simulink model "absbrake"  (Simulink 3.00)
settings: Solver=ode45  SolverMode=SingleTasking  StartTime=0.0  StopTime=25  MaxStep=.01  RelTol=1e-3  AbsTol=1e-6
PreLoadFcn:
  | absdata
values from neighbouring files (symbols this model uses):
  ctrl = 1    [absdata.m]
  g = 32.18    [absdata.m]    (also in f14dat.m = 32.2; watergui.m = locdrawwater(hilim, lolim, inflow, outflow, area); watersfun.m = get(ax,'UserData'))
  I = 5    [absdata.m]
  Kf = 1    [absdata.m]    (also in f14dat.m = -1.746; f14def.m = -1.746)
  m = 50    [absdata.m]    (also in rss.m = 1)
  mu = [0 .4 .8 .97 1.0 .98 .96 .94 .92 .9 .88 .855 .83 .81 .79 .77 .75 .73 .72 .71 .7]    [absdata.m]
  PBmax = 1500    [absdata.m]
  Rr = 15/12    (= 1.25)    [absdata.m]
  slip = (0:.05:1.0)    [absdata.m]
  TB = 0.01    [absdata.m]
  v0 = 88    [absdata.m]

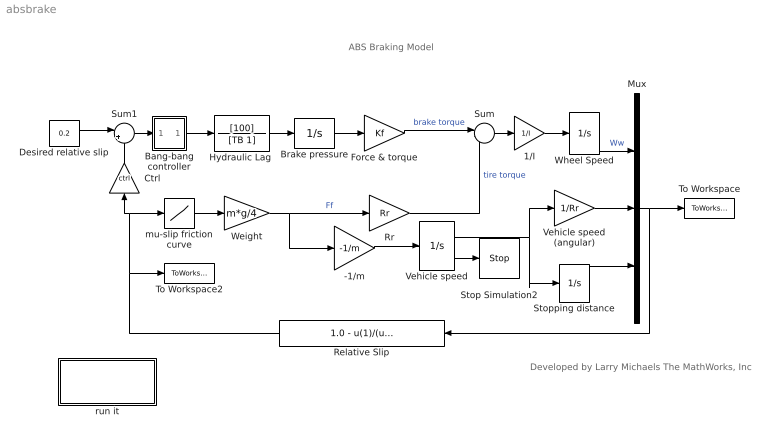
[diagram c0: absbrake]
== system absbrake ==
  note: ABS Braking Model
  note: Developed by Larry Michaels The MathWorks, Inc
  -1/m : Gain  Gain=-1/m  SaturateOnIntegerOverflow=on
  1/I : Gain  Gain=1/I  SaturateOnIntegerOverflow=on
  Bang-bang controller : Subsystem
  Brake pressure : Integrator  ExternalReset=none  InitialConditionSource=internal  InitialCondition=0  LimitOutput=on  UpperSaturationLimit=PBmax  LowerSaturationLimit=0  ShowSaturationPort=off  ShowStatePort=off  AbsoluteTolerance=auto
  Ctrl : Gain  Orientation=up  Gain=ctrl  SaturateOnIntegerOverflow=on
  Desired relative slip : Constant  Value=0.2
  Force & torque : Gain  Gain=Kf  SaturateOnIntegerOverflow=on
  "Hydraulic Lag " : TransferFcn  Numerator=[100]  Denominator=[TB 1]
  Mux : Mux  Inputs=3
  Relative Slip : Fcn  Orientation=left  Expr=1.0 - u(1)/(u(2) + (u(2)==0)*eps)
  Rr : Gain  Gain=Rr  SaturateOnIntegerOverflow=on
  Stop Simulation2 : Stop
  Stopping distance : Integrator  ExternalReset=none  InitialConditionSource=internal  InitialCondition=0  LimitOutput=off  UpperSaturationLimit=1000  LowerSaturationLimit=0  ShowSaturationPort=off  ShowStatePort=off  AbsoluteTolerance=auto
  Sum : Sum  Inputs=|-+  SaturateOnIntegerOverflow=on
  Sum1 : Sum  Inputs=|+-  SaturateOnIntegerOverflow=on
  To Workspace : ToWorkspace  VariableName=yout  SampleTime=0  SaveFormat=Matrix
  To Workspace2 : ToWorkspace  VariableName=slp  SampleTime=0  SaveFormat=Matrix
  Vehicle speed : Integrator  ExternalReset=none  InitialConditionSource=internal  InitialCondition=v0  LimitOutput=on  UpperSaturationLimit=1000  LowerSaturationLimit=0  ShowSaturationPort=on  ShowStatePort=off  AbsoluteTolerance=auto
  Vehicle speed (angular) : Gain  Gain=1/Rr  SaturateOnIntegerOverflow=on
  Weight : Gain  Gain=m*g/4  SaturateOnIntegerOverflow=on
  Wheel Speed : Integrator  ExternalReset=none  InitialConditionSource=internal  InitialCondition=v0/Rr  LimitOutput=on  UpperSaturationLimit=1000  LowerSaturationLimit=0  ShowSaturationPort=off  ShowStatePort=off  AbsoluteTolerance=auto
  mu-slip friction curve : Lookup  InputValues=slip  OutputValues=mu
  run it : Subsystem
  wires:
  1/I/1 -> Wheel Speed/1
  Mux/1 -> To Workspace/1, Relative Slip/1
  Sum/1 -> 1/I/1
  Wheel Speed/1 -> Mux/1  "Ww"
  Vehicle speed (angular)/1 -> Mux/2
  Relative Slip/1 -> To Workspace2/1, mu-slip friction curve/1, Ctrl/1
  Rr/1 -> Sum/2  "tire torque"
  Force & torque/1 -> Sum/1  "brake torque"
  Stopping distance/1 -> Mux/3
  -1/m/1 -> Vehicle speed/1
  Vehicle speed/2 -> Stop Simulation2/1
  Vehicle speed/1 -> Vehicle speed (angular)/1, Stopping distance/1
  mu-slip friction curve/1 -> Weight/1
  Weight/1 -> -1/m/1, Rr/1  "Ff"
  Brake pressure/1 -> Force & torque/1
  Ctrl/1 -> Sum1/2
  Bang-bang controller/1(out_1) -> "Hydraulic Lag "/1
  "Hydraulic Lag "/1 -> Brake pressure/1
  Desired relative slip/1 -> Sum1/1
  Sum1/1 -> Bang-bang controller/1(in_1)

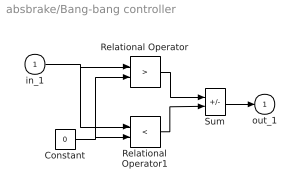
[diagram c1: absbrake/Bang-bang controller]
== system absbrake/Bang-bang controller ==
  in_1 : Inport  Port=1  PortWidth=-1  SampleTime=-1  DataType=auto
  Constant : Constant  Value=0
  Relational Operator : RelationalOperator  Operator=>
  Relational Operator1 : RelationalOperator  Operator=<
  Sum : Sum  Inputs=+-  SaturateOnIntegerOverflow=on
  out_1 : Outport  Port=1  InitialOutput=0
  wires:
  in_1/1 -> Relational Operator/1, Relational Operator1/1
  Constant/1 -> Relational Operator1/2, Relational Operator/2
  Relational Operator1/1 -> Sum/2
  Relational Operator/1 -> Sum/1
  Sum/1 -> out_1/1

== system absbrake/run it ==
